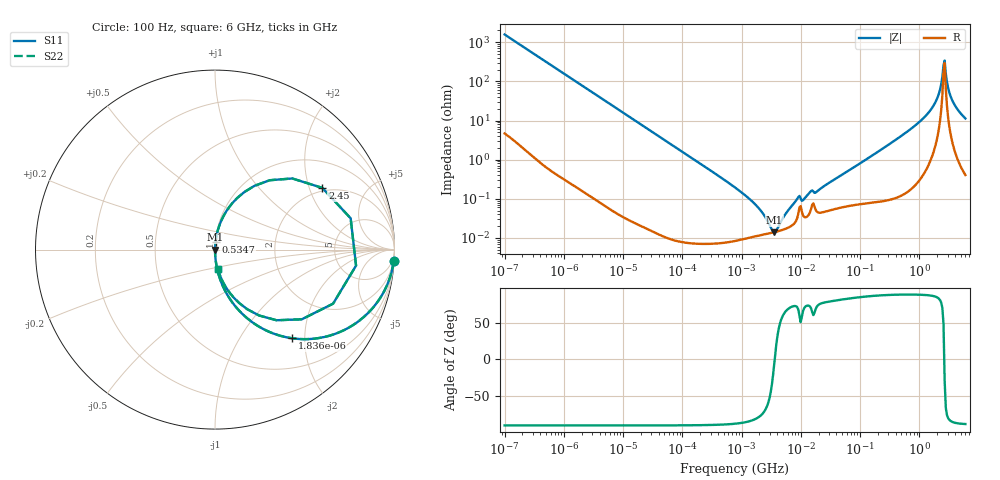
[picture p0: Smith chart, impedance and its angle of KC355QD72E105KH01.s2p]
!Murata Part Number: KC355QD72E105KH01
!These Parameters are Measured in Series Mode Connection
!Data Generated on Jun 19, 2026
!  o--ll--o
!Port1  Port2
!  o------o
!Operation Temp=25[degC], DC Bias Voltage=0[V]
!Freq. Start=100[Hz] Stop=6[GHz] 401[Steps]
# Hz S RI R 50
!Freq.(Hz) S11(Real) S11(Imag) S21(Real) S21(Imag) S12(Real) S12(Imag) S22(Real) S22(Imag)
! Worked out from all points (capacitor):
!   401 points, 100 Hz to 6 GHz, reference 50 ohm
!   read as one part in series: C = 1 uF near 109 Hz
!   lowest |Z| = 14.1 mohm at 3.55 MHz (marker M1)
!   series resonance near 3.622 MHz, so ESL is about 1.9 nH
!   S11 on the Smith chart (normalised r, x): 100 Hz: 1, -32; 1.836 kHz: 1.00, -1.73; 534.7 MHz: 1.00, +0.09; 2.45 GHz: 1.87, +2.46; 6 GHz: 1.01, -0.23
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100  0.9958 -0.0629  0.00416 0.0629  0.00416 0.0629  0.9958 -0.0629
548  0.8929 -0.3082  0.1071 0.3082  0.1071 0.3082  0.8929 -0.3082
1836  0.4284 -0.4938  0.5716 0.4938  0.5716 0.4938  0.4284 -0.4938
2008  0.3854 -0.4857  0.6146 0.4857  0.6146 0.4857  0.3854 -0.4857
5882  0.0687 -0.2519  0.9313 0.2519  0.9313 0.2519  0.0687 -0.2519
40335  0.00168 -0.0395  0.9983 0.0395  0.9983 0.0395  0.00168 -0.0395
774597  8.72e-05 -0.00194  0.9999 0.00194  0.9999 0.00194  8.72e-05 -0.00194
1896632  0.000114 -0.000593  0.9999 0.000593  0.9999 0.000593  0.000114 -0.000593
3549919  0.00014 -1.68e-05  0.9999 1.68e-05  0.9999 1.68e-05  0.00014 -1.68e-05
8692127  0.00032 0.000941  0.9997 -0.000941  0.9997 -0.000941  0.00032 0.000941
1.137099e7  0.000345 0.000932  0.9997 -0.000932  0.9997 -0.000932  0.000345 0.000932
1.555665e7  0.000702 0.00148  0.9993 -0.00148  0.9993 -0.00148  0.000702 0.00148
3.124326e8  0.00155 0.0248  0.9984 -0.0248  0.9984 -0.0248  0.00155 0.0248
5.346885e8  0.00317 0.0436  0.9968 -0.0436  0.9968 -0.0436  0.00317 0.0436
1.144649e9  0.0158 0.1083  0.9842 -0.1083  0.9842 -0.1083  0.0158 0.1083
1.791126e9  0.0775 0.2347  0.9225 -0.2347  0.9225 -0.2347  0.0775 0.2347
2.142435e9  0.2202 0.3554  0.7798 -0.3554  0.7798 -0.3554  0.2202 0.3554
2.450438e9  0.5981 0.3438  0.4019 -0.3438  0.4019 -0.3438  0.5981 0.3438
2.679998e9  0.7858 -0.0893  0.2142 0.0893  0.2142 0.0893  0.7858 -0.0893
3.065283e9  0.3427 -0.3937  0.6573 0.3937  0.6573 0.3937  0.3427 -0.3937
3.8344e9  0.0834 -0.2427  0.9166 0.2427  0.9166 0.2427  0.0834 -0.2427
6e9  0.0165 -0.1106  0.9835 0.1106  0.9835 0.1106  0.0165 -0.1106
